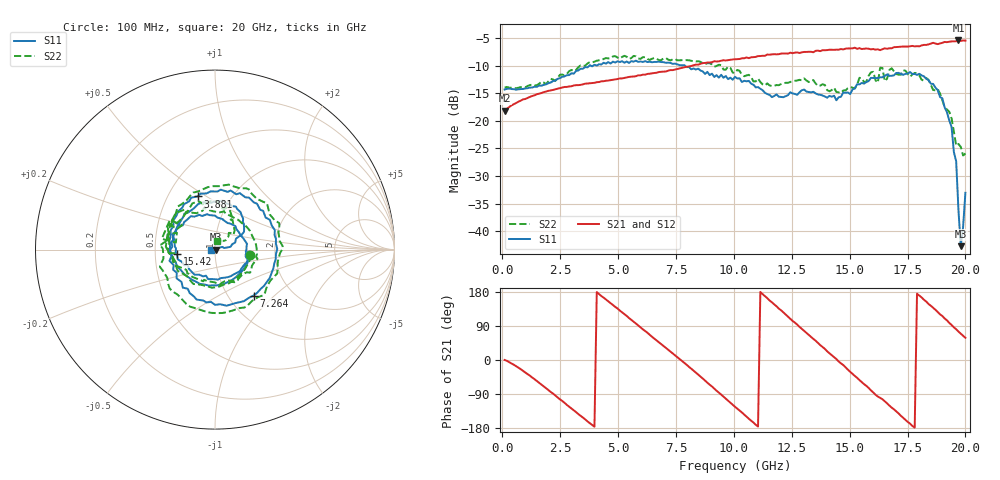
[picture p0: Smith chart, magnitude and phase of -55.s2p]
!Agilent Technologies,N5230C,MY49001569,A.09.33.09
!Agilent N5230C: A.09.33.09
!Date: Monday, July 27, 2015 12:37:58
!Correction: S11(Full 2 Port(1,2))
!S21(Full 2 Port(1,2))
!S12(Full 2 Port(1,2))
!S22(Full 2 Port(1,2))
!S2P File: Measurements: S11, S21, S12, S22:
# Hz S  dB  R 50
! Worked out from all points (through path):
!   201 points, 100 MHz to 20 GHz, reference 50 ohm
!   highest |S21| = -5.44 dB at 19.7 GHz (marker M1); lowest = -18.2 dB at 100 MHz (marker M2)
!   group delay of S21, straight-line fit = 144 ps
!   lowest |S11| = -42.7 dB at 19.8 GHz (marker M3), VSWR 1.01, Z = 50.7 - j0.0437 ohm
!   |S11| at or under -10 dB: start of sweep to 3.765 GHz; 3.814 GHz to 3.927 GHz (113 MHz wide, 2.92 % of centre); 7.884 GHz to end of sweep
!   |S22| runs from -26.3 to -8.2 dB; largest |S21 - S12| = 0.022
!   S11 on the Smith chart (normalised r, x): 100 MHz: 1.46, -0.09; 3.881 GHz: 0.70, +0.46; 7.264 GHz: 1.30, -0.75; 15.42 GHz: 0.65, -0.03; 20 GHz: 0.96, -0.00
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1e8  -14.33 -9.3  -18.17 0.1  -17.96 0.5  -13.98 -8.5
1.692e9  -13.64 -121.5  -14.97 -64.5  -14.95 -65.1  -12.91 -122.0
3.483e9  -10.57 127.9  -13.40 -152.0  -13.42 -152.5  -10.06 127.0
3.881e9  -10.13 108.2  -13.17 -171.3  -13.13 -171.4  -9.44 106.4
5.672e9  -9.28 22.8  -11.98 100.9  -11.95 100.5  -8.24 22.4
6.7665e9  -9.28 -27.4  -11.16 46.9  -11.15 46.0  -9.02 -28.9
7.264e9  -9.52 -50.0  -10.81 22.3  -10.83 21.3  -9.06 -53.9
8.458e9  -10.56 -110.2  -9.83 -38.4  -9.81 -39.3  -9.20 -113.6
1.005e10  -12.03 160.0  -8.85 -123.5  -8.87 -124.5  -11.34 157.9
1.1443e10  -15.15 75.0  -7.99 163.3  -8.13 162.3  -13.22 76.9
1.2438e10  -14.84 10.3  -7.66 108.8  -7.77 108.6  -12.98 14.9
1.3433e10  -14.74 -41.1  -7.58 55.7  -7.46 55.0  -12.63 -33.4
1.43285e10  -15.45 -103.1  -7.15 7.6  -7.01 6.4  -14.02 -82.9
1.5423e10  -13.41 -173.2  -6.83 -52.9  -6.96 -53.5  -12.21 -159.8
1.67165e10  -11.87 125.1  -6.86 -120.2  -6.85 -120.8  -10.79 151.2
1.801e10  -11.49 64.1  -6.51 170.0  -6.34 169.4  -11.80 85.3
1.9005e10  -15.93 29.0  -5.87 116.1  -5.74 113.8  -16.31 44.4
1.9403e10  -21.11 10.1  -5.62 92.5  -5.65 91.2  -19.57 44.4
1.9602e10  -27.34 20.6  -5.59 81.1  -5.61 80.3  -24.51 50.8
1.97015e10  -36.27 28.5  -5.44 74.9  -5.44 73.3  -24.20 69.3
1.9801e10  -42.72 -3.4  -5.53 69.3  -5.51 68.0  -24.74 72.3
2e10  -33.05 -177.6  -5.47 58.5  -5.51 56.4  -25.92 75.1
